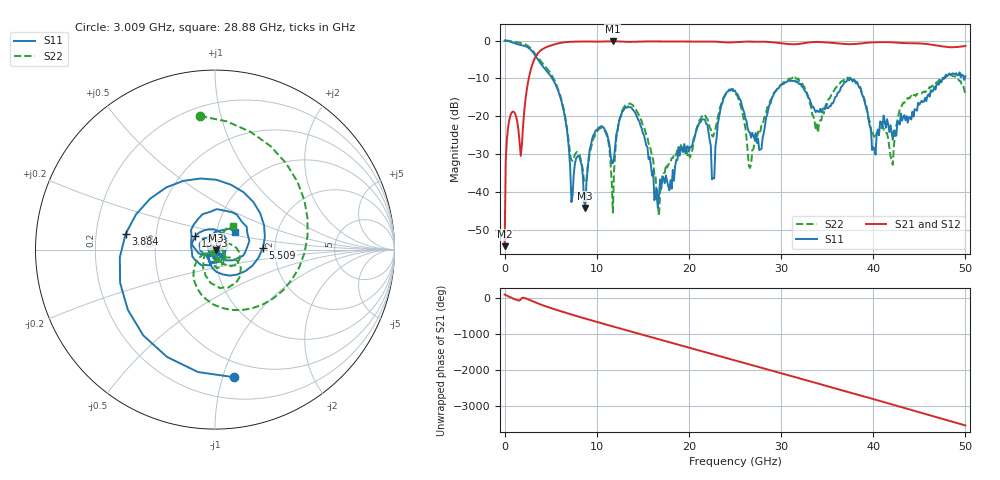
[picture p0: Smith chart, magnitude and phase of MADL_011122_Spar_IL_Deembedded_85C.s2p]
#	HZ	S	DB	R	50
!Frequency	S11 (dB)	S11-Ang	S21 Deemb (dB)	S21-Ang	S12 Deemb (dB)	S12-Ang	S22 (dB)	S22-Ang
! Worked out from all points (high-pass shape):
!   401 points, 10 MHz to 50 GHz, reference 50 ohm
!   highest |S21| = -0.18 dB at 11.76 GHz (marker M1); lowest = -54.3 dB at 10 MHz (marker M2)
!   |S21| within 3 dB of the highest: 3.692 GHz to end of sweep
!   lowest |S11| = -44.3 dB at 8.758 GHz (marker M3), VSWR 1.01, Z = 50.5 - j0.39 ohm
!   |S11| at or under -10 dB: 5.181 GHz to 47.58 GHz (42.4 GHz wide, 161 % of centre); 47.74235 GHz to 47.75177 GHz (9.416 MHz wide, 0.0197 % of centre); 49.83052 GHz to 49.92712 GHz (96.6 MHz wide, 0.194 % of centre)
!   |S22| runs from -46.4 to 0.0 dB; largest |S21 - S12| = 0.0086
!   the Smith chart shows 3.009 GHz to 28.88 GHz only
!   S11 on the Smith chart (normalised r, x): 3.009 GHz: 0.37, -1.09; 3.884 GHz: 0.33, +0.08; 5.509 GHz: 1.73, +0.03; 13.63 GHz: 0.79, +0.12; 28.88 GHz: 1.23, +0.25
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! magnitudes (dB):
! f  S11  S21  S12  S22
! 10 MHz  0.0  -54.3  -53.6  0.0
! 509.9 MHz  -0.2  -21.1  -21.1  -0.1
! 1.76 GHz  -1.2  -30.5  -30.5  -0.6
! 3.009 GHz  -2.9  -6.4  -6.4  -2.5
! 3.884 GHz  -5.9  -2.7  -2.7  -5.3
! 5.509 GHz  -11.5  -0.9  -0.9  -11.0
! 7.259 GHz  -42.7  -0.3  -0.3  -31.5
! 8.383 GHz  -33.0  -0.2  -0.2  -32.8
! 8.758 GHz  -44.3  -0.2  -0.2  -37.2
! 10.51 GHz  -22.6  -0.3  -0.3  -23.0
! 11.76 GHz  -32.4  -0.2  -0.2  -45.5
! 13.63 GHz  -17.6  -0.3  -0.3  -16.6
! 16.76 GHz  -40.9  -0.2  -0.2  -46.4
! 21.51 GHz  -20.8  -0.3  -0.3  -19.7
! 22.76 GHz  -36.4  -0.3  -0.3  -24.4
! 25 GHz  -13.2  -0.4  -0.4  -13.7
! 26.63 GHz  -24.3  -0.3  -0.3  -33.7
! 28.88 GHz  -16.5  -0.4  -0.4  -15.7
! 33.38 GHz  -17.5  -0.4  -0.4  -19.6
! 37.63 GHz  -10.1  -1.0  -1.0  -10.2
! 41.75 GHz  -24.2  -0.4  -0.5  -28.3
! 50 GHz  -9.4  -1.4  -1.4  -14.0
